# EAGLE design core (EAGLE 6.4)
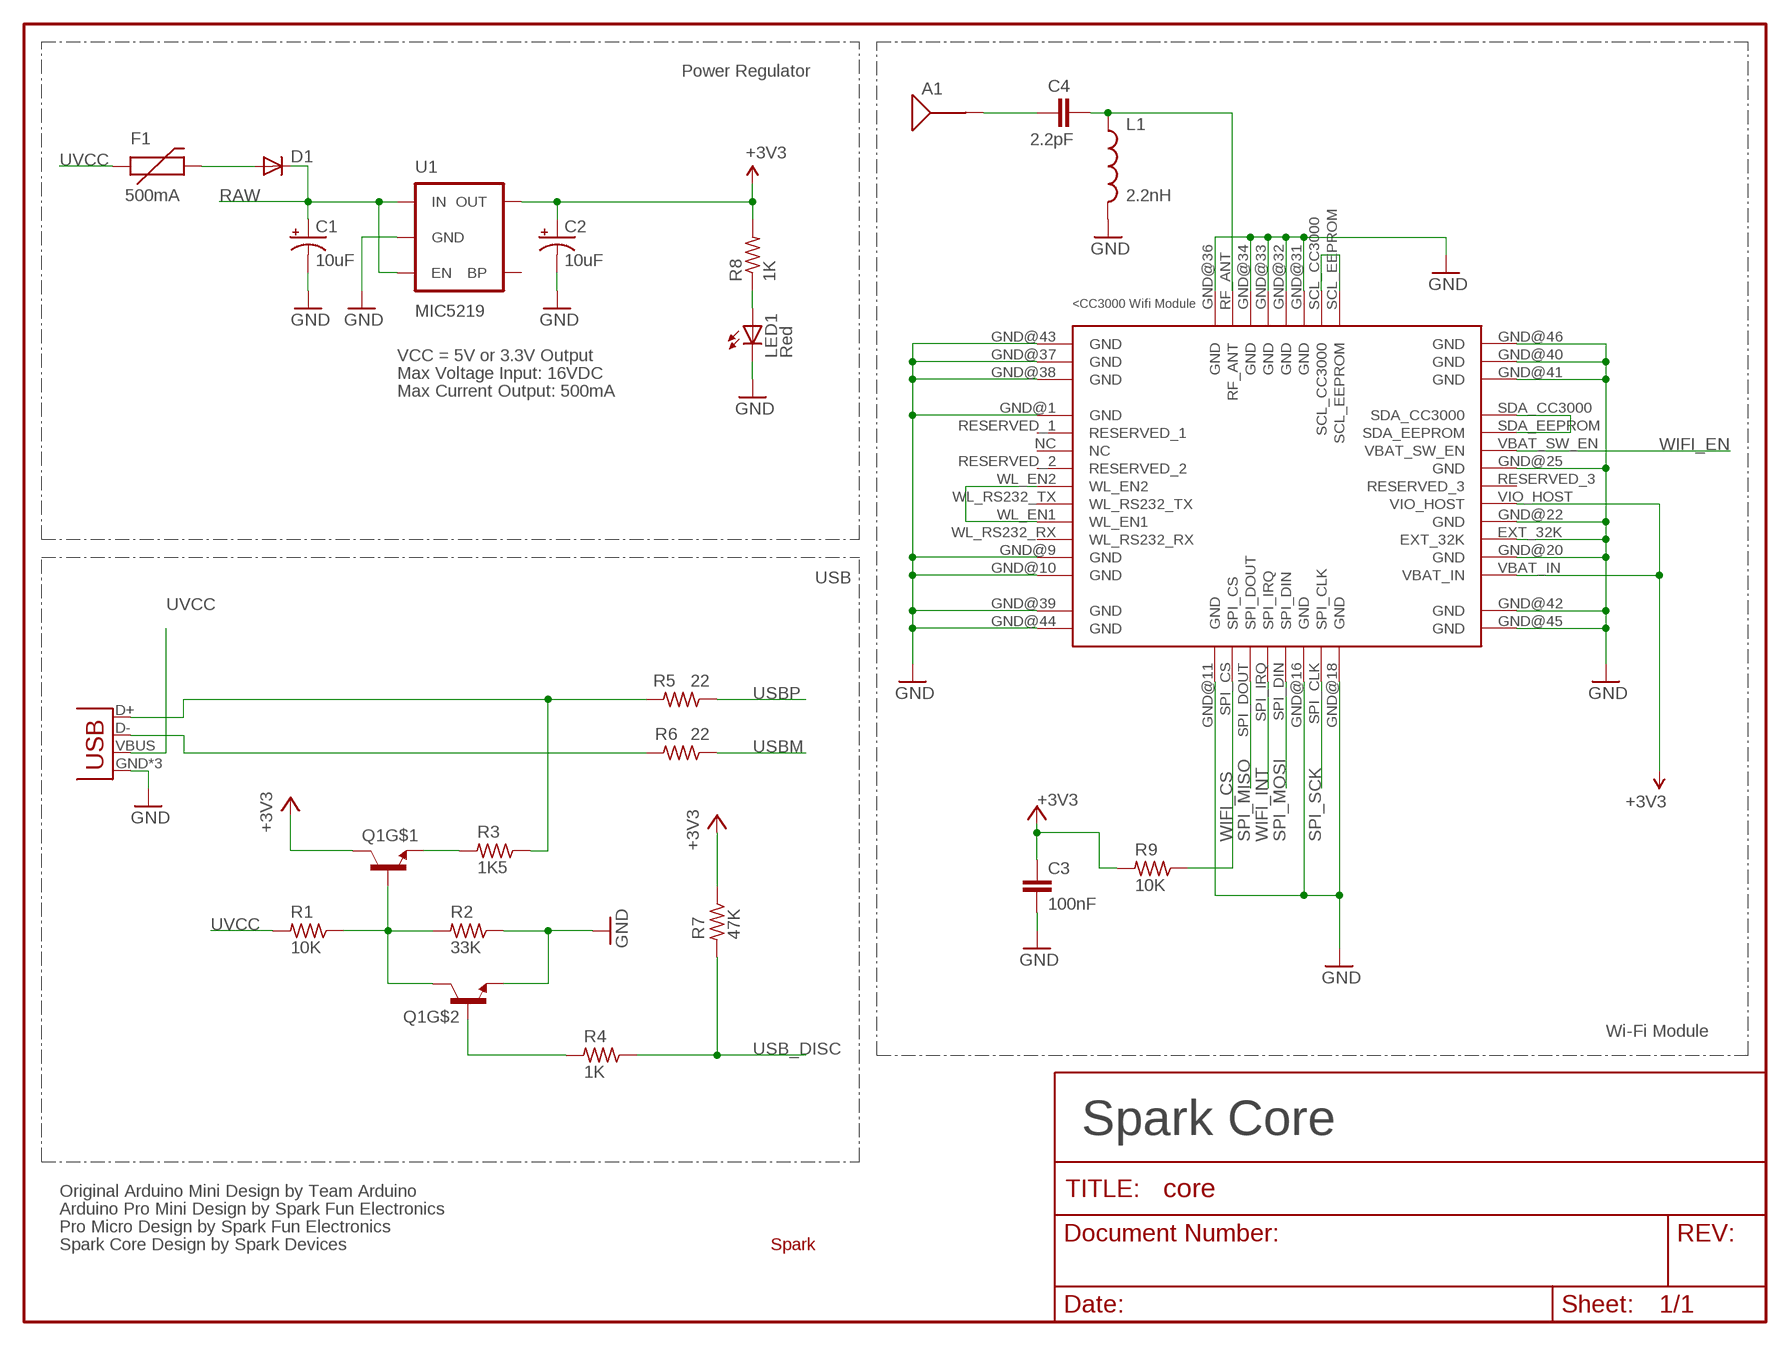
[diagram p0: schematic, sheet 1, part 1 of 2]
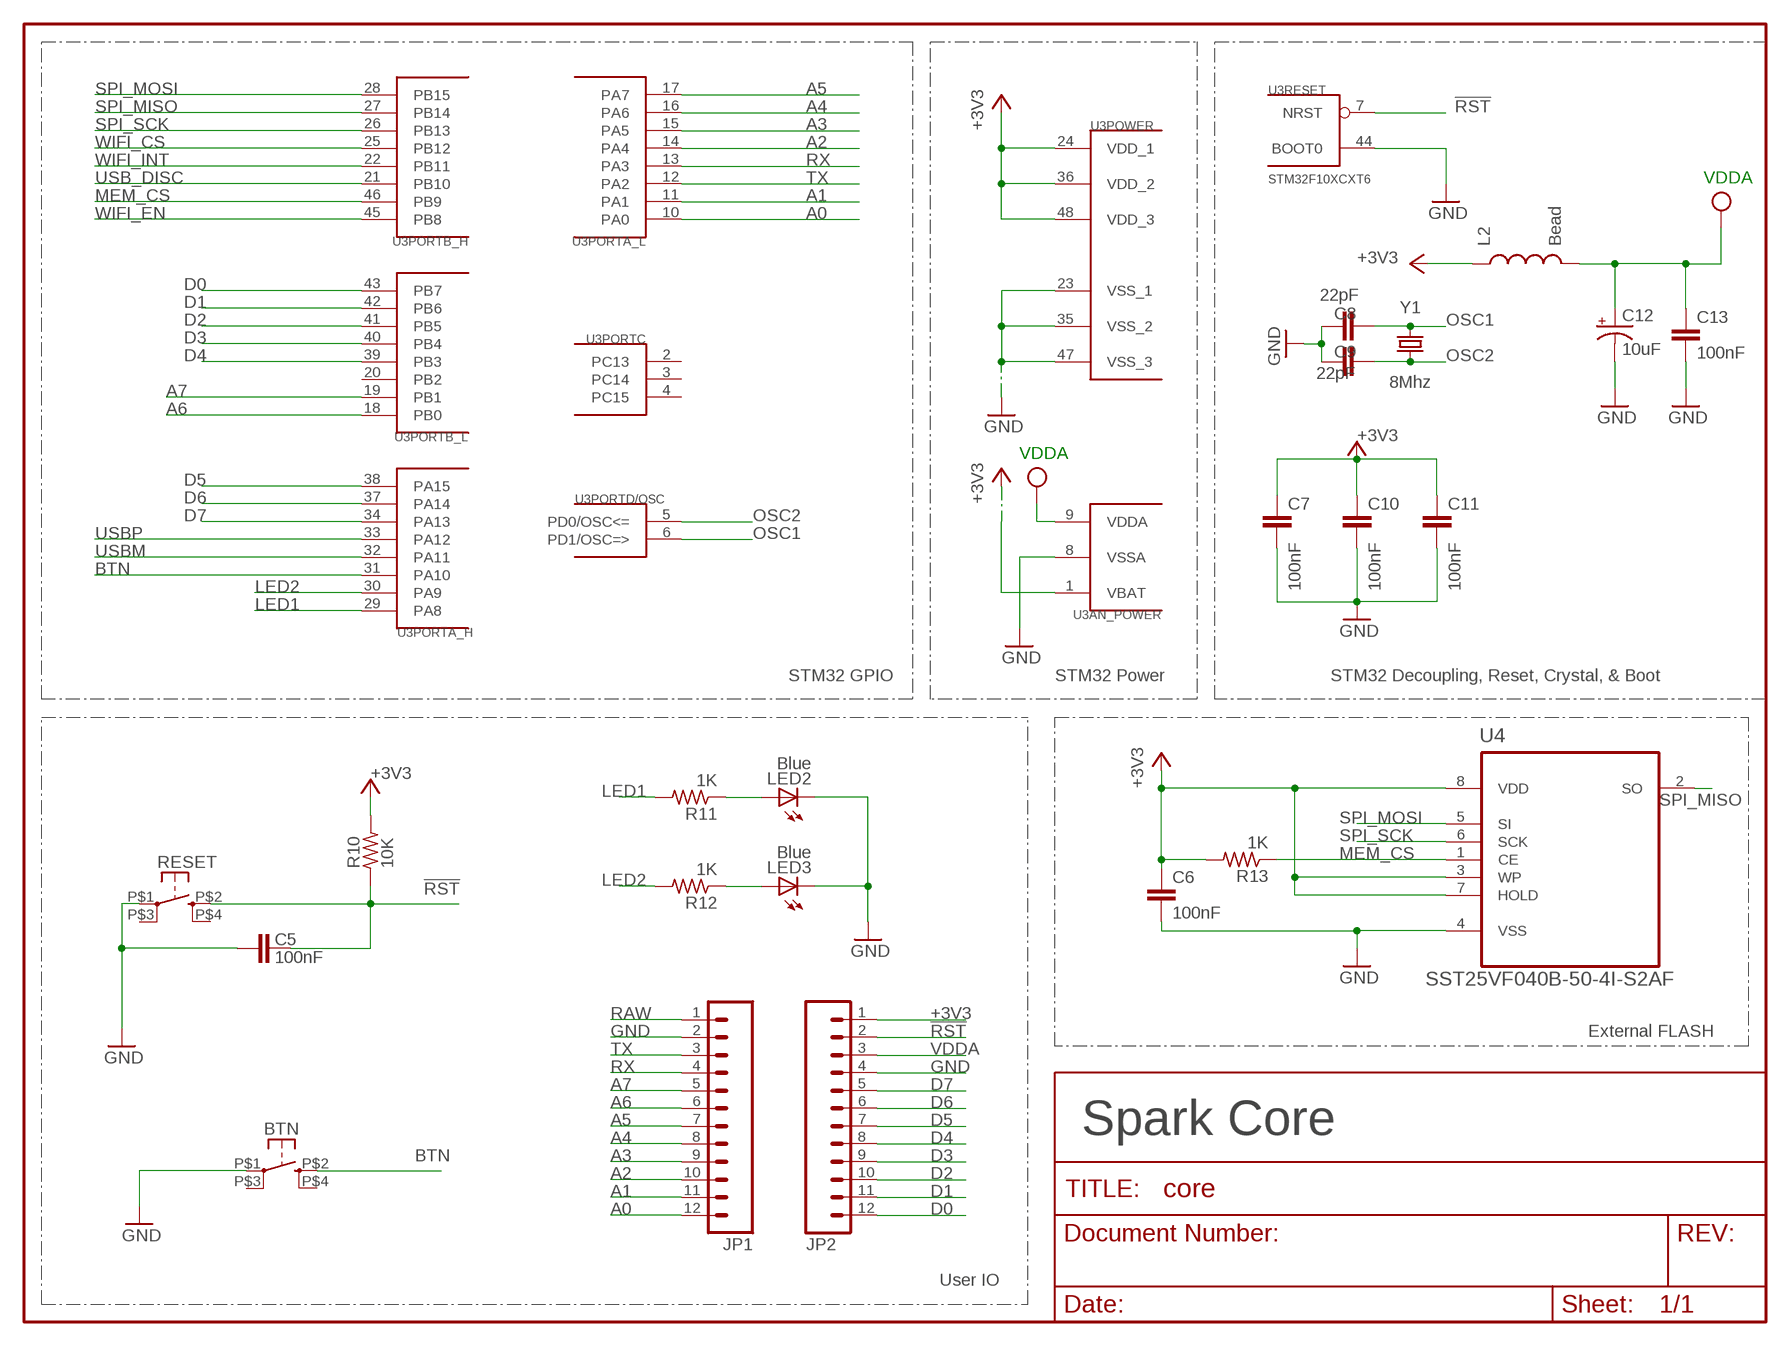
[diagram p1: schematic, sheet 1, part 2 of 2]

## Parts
A1  ANTENNA2SMD5  [ANTENNA-CHIP5]
BTN  KMR211GLFS  BUTTON-KMR241GLFS  [PUSHBUTTON-KMR241GLFS]
C1  10uF  CAP_POL1206  [EIA3216]
C2  10uF  CAP_POL1206  [EIA3216]
C3  100nF  C-EUC0603  [C0603]
C4  2.2pF  C-EUC0603  [C0603]
C5  100nF  C-EUC0603  [C0603]
C6  100nF  C-EUC0603  [C0603]
C7  100nF  C-EUC0603  [C0603]
C8  22pF  C-EUC0603  [C0603]
C9  22pF  C-EUC0603  [C0603]
C10  100nF  C-EUC0603  [C0603]
C11  100nF  C-EUC0603  [C0603]
C12  10uF  CAP_POL1206  [EIA3216]
C13  100nF  C-EUC0603  [C0603]
D1  DIODESOD  [SOD-323]
F1  500mA  PTCSMD  [PTC-1206]
JP1  M12PTH  [1X12]
JP2  M12PTH  [1X12]
L1  2.2nH  INDUCTOR0603  [0603]
L2  Bead  INDUCTOR0603  [0603]
LED1  Red  LED0603  [LED-0603]
LED2  Blue  LED0603  [LED-0603]
LED3  Blue  LED0603  [LED-0603]
Q1  MMDT3904  [SOT363]
R1  10K  R-US_R0603  [R0603]
R2  33K  R-US_R0603  [R0603]
R3  1K5  R-US_R0603  [R0603]
R4  1K  R-US_R0603  [R0603]
R5  22  R-US_R0603  [R0603]
R6  22  R-US_R0603  [R0603]
R7  47K  R-US_R0603  [R0603]
R8  1K  R-US_R0603  [R0603]
R9  10K  R-US_R0603  [R0603]
R10  10K  R-US_R0603  [R0603]
R11  1K  R-US_R0603  [R0603]
R12  1K  R-US_R0603  [R0603]
R13  1K  R-US_R0603  [R0603]
RESET  KMR211GLFS  BUTTON-KMR241GLFS  [PUSHBUTTON-KMR241GLFS]
U1  MIC5219  V_REG_LDOSMD  [SOT23-5]
U2  CC3000  [CC3000]
U3  STM32F10XCXT6  [TQFP48]
U4  SST25VF040B-50-4I-S2AF  [SOIC127P790X216-8N]
U$1  SPARK_LOGO2  [SPARK_LOGO2]
X1  USB-MICROB  USBUSB-MICROB-ALIGN  [USB-MICROB-ALIGN]
Y1  8Mhz  CRYSTAL5X3  [CRYSTAL-SMD-5X3]

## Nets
!RST: C5.2 JP2.2 R10.1 RESET.P$2 U3.7(RESET:NRST)
+3V3: C2.A(+) C3.1 C6.1 C7.1 C10.1 C11.1 JP2.1 L2.1 Q1.3(C) R7.1 R8.2 R9.2 R10.2 R13.2 U1.5(OUT) U2.VBAT_IN U2.VIO_HOST U3.1(AN_POWER:VBAT) U3.24(POWER:VDD_1) U3.36(POWER:VDD_2) U3.48(POWER:VDD_3) U4.3(WP) U4.7(HOLD) U4.8(VDD)
A0: JP1.12 U3.10(PORTA_L:PA0)
A1: JP1.11 U3.11(PORTA_L:PA1)
A2: JP1.10 U3.14(PORTA_L:PA4)
A3: JP1.9 U3.15(PORTA_L:PA5)
A4: JP1.8 U3.16(PORTA_L:PA6)
A5: JP1.7 U3.17(PORTA_L:PA7)
A6: JP1.6 U3.18(PORTB_L:PB0)
A7: JP1.5 U3.19(PORTB_L:PB1)
BTN: BTN.P$2 U3.31(PORTA_H:PA10)
D0: JP2.12 U3.43(PORTB_L:PB7)
D1: JP2.11 U3.42(PORTB_L:PB6)
D2: JP2.10 U3.41(PORTB_L:PB5)
D3: JP2.9 U3.40(PORTB_L:PB4)
D4: JP2.8 U3.39(PORTB_L:PB3)
D5: JP2.7 U3.38(PORTA_H:PA15)
D6: JP2.6 U3.37(PORTA_H:PA14)
D7: JP2.5 U3.34(PORTA_H:PA13)
GND [vcc]: BTN.P$1 C1.C(-) C2.C(-) C3.2 C5.1 C6.2 C7.2 C8.2 C9.2 C10.2 C11.2 C12.C(-) C13.2 JP1.2 JP2.4 L1.2 LED1.C LED2.C LED3.C Q1.1(E) R2.1 RESET.P$1 U1.2(GND) U2.EXT_32K U2.GND@1(GND) U2.GND@9(GND) U2.GND@10(GND) U2.GND@11(GND) U2.GND@16(GND) U2.GND@18(GND) U2.GND@20(GND) U2.GND@22(GND) U2.GND@25(GND) U2.GND@31(GND) U2.GND@32(GND) U2.GND@33(GND) U2.GND@34(GND) U2.GND@36(GND) U2.GND@37(GND) U2.GND@38(GND) U2.GND@39(GND) U2.GND@40(GND) U2.GND@41(GND) U2.GND@42(GND) U2.GND@43(GND) U2.GND@44(GND) U2.GND@45(GND) U2.GND@46(GND) U3.8(AN_POWER:VSSA) U3.23(POWER:VSS_1) U3.35(POWER:VSS_2) U3.44(RESET:BOOT0) U3.47(POWER:VSS_3) U4.4(VSS) X1.GND X1.MT1(GND) X1.MT2(GND)
LED1: R11.2 U3.29(PORTA_H:PA8)
LED2: R12.2 U3.30(PORTA_H:PA9)
MEM_CS: R13.1 U3.46(PORTB_H:PB9) U4.1(CE)
N$1: R3.1 R5.2 X1.D+
N$2: LED2.A R11.1
N$3: D1.2(A) F1.2
N$4: C4.2 L1.1 U2.RF_ANT
N$5: A1.FEED(SIGNAL) C4.1
N$6: R6.2 X1.D-
N$7: U2.SCL_CC3000 U2.SCL_EEPROM
N$8: Q1.2(B) R4.2
N$9: U2.WL_EN1 U2.WL_EN2
N$10: LED3.A R12.1
N$13: Q1.5(B) Q1.6(C) R1.1 R2.2
N$15: U2.SDA_CC3000 U2.SDA_EEPROM
N$16: Q1.4(E) R3.2
N$38: LED1.A R8.1
OSC1: C8.1 U3.6(PORTD/OSC:PD1/OSC=>) Y1.3
OSC2: C9.1 U3.5(PORTD/OSC:PD0/OSC<=) Y1.1
RAW [vcc]: C1.A(+) D1.1(C) JP1.1 U1.1(IN) U1.3(EN)
RX: JP1.4 U3.13(PORTA_L:PA3)
SPI_MISO: U2.SPI_DOUT U3.27(PORTB_H:PB14) U4.2(SO)
SPI_MOSI: U2.SPI_DIN U3.28(PORTB_H:PB15) U4.5(SI)
SPI_SCK: U2.SPI_CLK U3.26(PORTB_H:PB13) U4.6(SCK)
TX: JP1.3 U3.12(PORTA_L:PA2)
USB_DISC: R4.1 R7.2 U3.21(PORTB_H:PB10)
USBM: R6.1 U3.32(PORTA_H:PA11)
USBP: R5.1 U3.33(PORTA_H:PA12)
UVCC: F1.1 R1.2 X1.VBUS
VDDA: C12.A(+) C13.1 JP2.3 L2.2 U3.9(AN_POWER:VDDA) ; supply symbol labelled VCC
WIFI_CS: R9.1 U2.SPI_CS U3.25(PORTB_H:PB12)
WIFI_EN: U2.VBAT_SW_EN U3.45(PORTB_H:PB8)
WIFI_INT: U2.SPI_IRQ U3.22(PORTB_H:PB11)
Unconnected: BTN.P$3 BTN.P$4 RESET.P$3 RESET.P$4 U1.4(BP) U2.NC U2.RESERVED_1 U2.RESERVED_2 U2.RESERVED_3 U2.WL_RS232_RX U2.WL_RS232_TX U3.2(PORTC:PC13) U3.3(PORTC:PC14) U3.4(PORTC:PC15) U3.20(PORTB_L:PB2)

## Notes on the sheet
- Power Regulator
- VDDA
- VCC = 5V or 3.3V Output
- Max Voltage Input: 16VDC
- Max Current Output: 500mA
- VDDA
- USB
- STM32 GPIO | STM32 Power | STM32 Decoupling, Reset, Crystal, & Boot
- Wi-Fi Module | External FLASH
- Spark Core | Spark Core
- Original Arduino Mini Design by Team Arduino
- Arduino Pro Mini Design by Spark Fun Electronics
- Pro Micro Design by Spark Fun Electronics
- Spark Core Design by Spark Devices
- User IO

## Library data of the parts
A1 = SparkFun-RF:ANTENNA2: Chip antenna
BTN RESET = okie:BUTTON-KMR241GLFS
C1 C2 C12 = SparkFun:CAP_POL: Capacitor Polarized
C3-C11 C13 = rcl:C-EU: CAPACITOR, European symbol
D1 = SparkFun:DIODE: Diode
F1 = SparkFun:PTC: Resettable Fuse PTC
JP1 JP2 = SparkFun:M12: Header 12 Standard 12-pin 0.1" header. Use with straight break away headers (SKU : PRT-00116), right angle break away headers (PRT-00553), swiss pins (PRT-00743), machine pins (PRT-00117), and female headers (PRT-00115).
L1 L2 = SparkFun-Passives:INDUCTOR: Inductors
LED1-LED3 = SparkFun:LED: LEDs
Q1 = SparkFun-DiscreteSemi:MMDT3904: Dual NPN transistor
R1-R13 = rcl:R-US_: RESISTOR, American symbol
U1 = SparkFun:V_REG_LDO: Voltage Regulator LDO Standard 150mA LDO voltage regulator in SOT-23 layout. Micrel part MIC5205. BP (by-pass) pin is used to lower output noise with 470pF cap.
U2 = CC3000:CC3000
U3 = stm32:STM32F10XCXT6: ST STM32F101/103 48pin LQFP
U4 = Silicon_Storage_Tech_By_element14_Batch_1:SST25VF040B-50-4I-S2AF: 4 Mbit SPI Serial Flash; MPN: SST25VF040B-50-4I-S2AF; OC_FARNELL: 1368690; OC_NEWARK: -; PACKAGE: SOIC-8; SUPPLIER: SILICON STORAGE TECHNOLOGY
U$1 = Spark:SPARK_LOGO2
X1 = Spark:USB: USB Connectors USB-B-PTH is fully proven SKU : PRT-00139/CONN-08278 USB-miniB is fully proven SKU : PRT-00587 USB-A-PCB is untested. USB-A-H is throughly reviewed, but untested. Spark Fun Electronics SKU : PRT-00437 USB-B-SMT is throughly reviewed, but untested. Needs silkscreen touching up.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
Y1 = SparkFun:CRYSTAL: Crystals

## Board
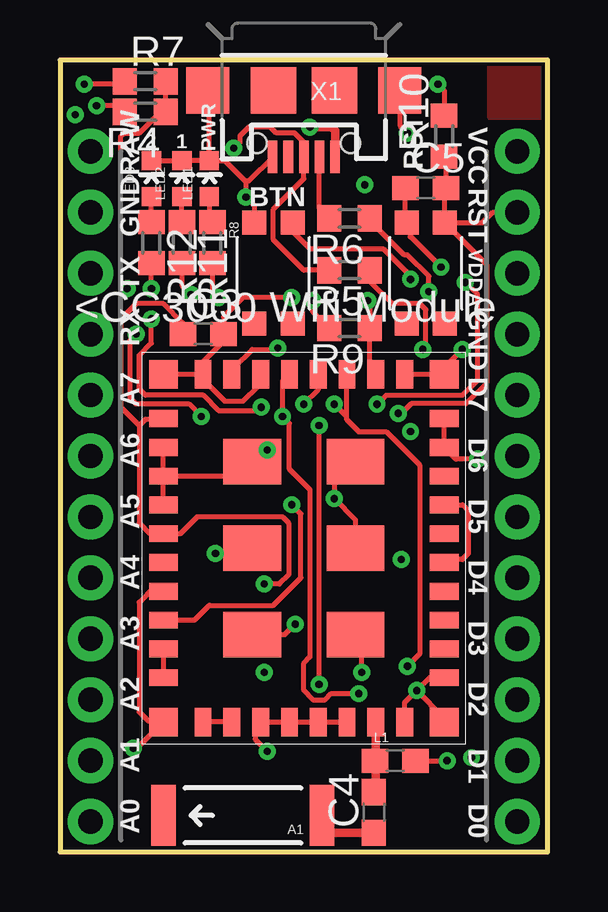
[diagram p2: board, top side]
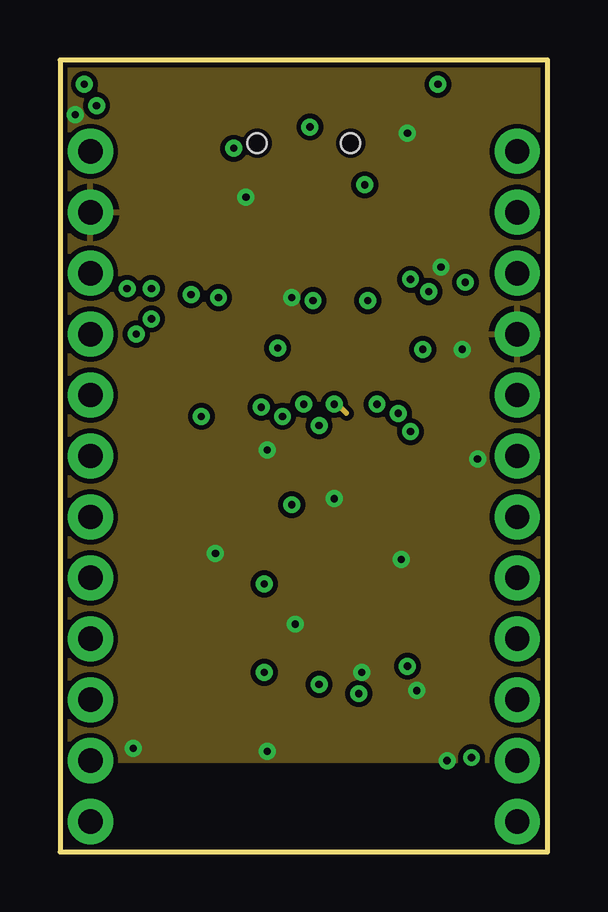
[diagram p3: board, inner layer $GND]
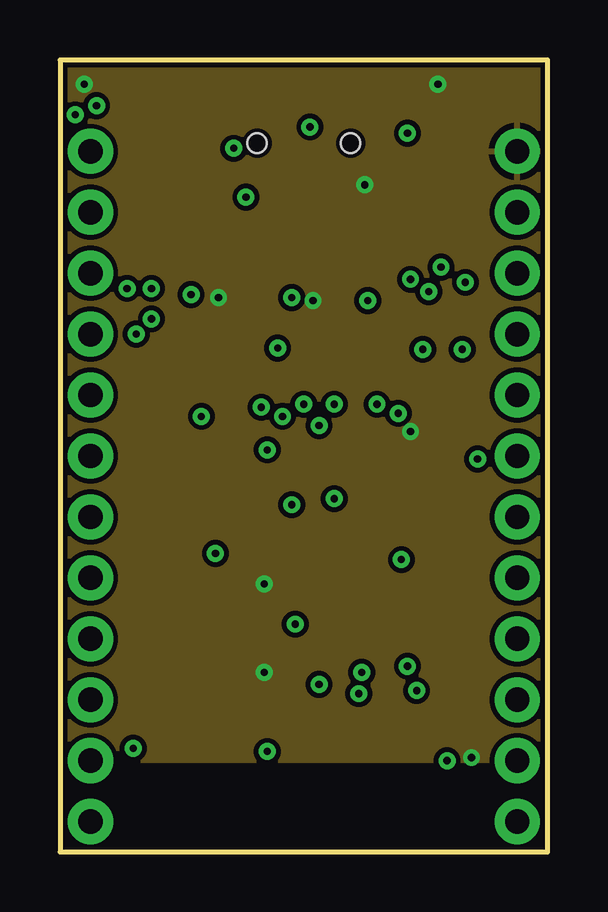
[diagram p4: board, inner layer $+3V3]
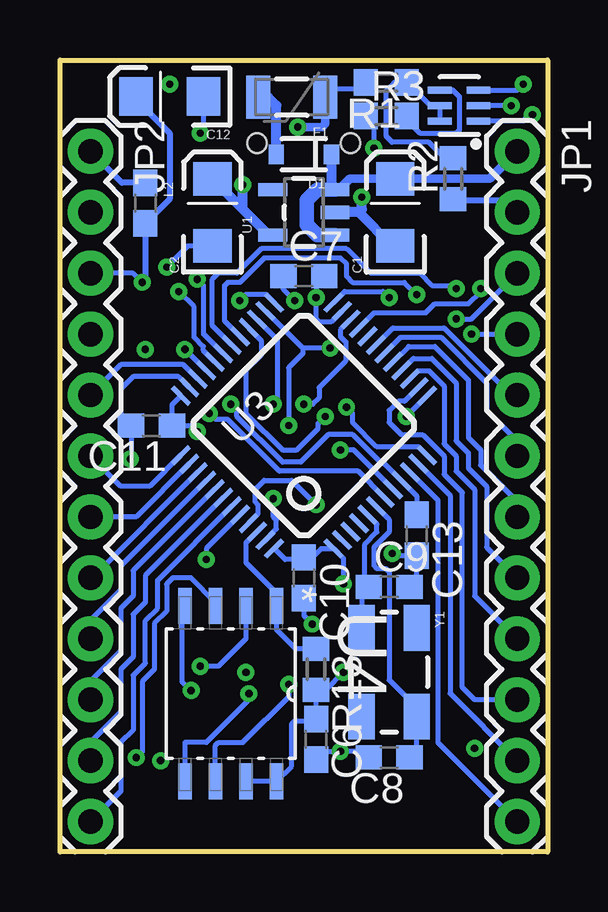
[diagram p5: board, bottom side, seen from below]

Size 20.32 x 33.02 mm. Coordinates in mm from the lower left corner, seen from the top.
Outline: 0,33.02 0,0 20.32,0 20.32,33.02 0,33.02
Copper layers (1+2*15+16): Top 0.035mm / dielectric 1.5mm / $GND 0.035mm / dielectric 0.15mm / $+3V3 0.035mm / dielectric 0.2mm / Bottom 0.035mm
Design rules "default *": minimum track width 6mil, minimum drill 0.3mm, track to track 6mil, track to pad 6mil, pad to pad 6mil, via to via 6mil, smd to smd 6mil, copper to edge 6mil, drill to drill 6mil, minimum pad ring 12mil, minimum via ring 8mil, stop-mask expansion 4mil, vias tented up to drill 20mil, thermal gap 10mil

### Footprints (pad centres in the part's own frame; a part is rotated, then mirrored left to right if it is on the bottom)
ANTENNA-CHIP5 = smd 1.016 x 2.54: FEED -3.302,0; NC 3.302,0
PUSHBUTTON-KMR241GLFS = smd 1 x 1: P$1 2.1,0.8; P$2 2.1,-0.8; P$3 -2.1,0.8; P$4 -2.1,-0.8
EIA3216 = smd 1.4 x 1.6: A 1.4,0; C -1.4,0
C0603 = smd 1.1 x 1: 1 -0.85,0; 2 0.85,0
SOD-323 = smd 0.63 x 0.83: 1 -1.15,0; 2 1.15,0
PTC-1206 = smd 1 x 1.8: 1 -1.4,0; 2 1.4,0
1X12 = drill 1.016 pad 1.88: 1 0,0; 2 2.54,0; 3 5.08,0; 4 7.62,0; 5 10.16,0; 6 12.7,0; 7 15.24,0; 8 17.78,0; 9 20.32,0; 10 22.86,0; 11 25.4,0; 12 27.94,0
0603 = smd 1.1 x 1: 1 -0.85,0; 2 0.85,0
LED-0603 = smd 0.8 x 0.8: A 0,-0.75; C 0,0.75
SOT363 = smd 0.3 x 0.99: 1 -0.65,-0.8; 2 0,-0.8; 3 0.65,-0.8; 4 0.65,0.81; 5 0,0.81; 6 -0.65,0.81
R0603 = smd 1 x 1.1: 1 -0.85,0; 2 0.85,0
SOT23-5 = smd 0.55 x 1.2: 1 -0.95,-1.3; 2 0,-1.3; 3 0.95,-1.3; 4 0.95,1.3; 5 -0.95,1.3
CC3000 = smd 1.2 x 0.7: EXT_32K 5.85,-2.97; GND@1 -5.85,5.43; GND@9 -5.85,-4.17; GND@10 -5.85,-5.37; GND@20 5.85,-4.17; GND@22 5.85,-1.77; GND@25 5.85,1.83; NC -5.85,3.03; RESERVED_1 -5.85,4.23; RESERVED_2 -5.85,1.83; RESERVED_3 5.85,0.63; SDA_CC3000 5.85,5.43; SDA_EEPROM 5.85,4.23; VBAT_IN 5.85,-5.37; VBAT_SW_EN 5.85,3.03; VIO_HOST 5.85,-0.57; WL_EN1 -5.85,-1.77; WL_EN2 -5.85,0.63; WL_RS232_RX -5.85,-2.97; WL_RS232_TX -5.85,-0.57 | smd 0.7 x 1.2: GND@11 -4.2,-7.22; GND@16 1.8,-7.22; GND@18 4.2,-7.22; GND@31 1.8,7.28; GND@32 0.6,7.28; GND@33 -0.6,7.28; GND@34 -1.8,7.28; GND@36 -4.2,7.28; RF_ANT -3,7.28; SCL_CC3000 3,7.28; SCL_EEPROM 4.2,7.28; SPI_CLK 3,-7.22; SPI_CS -3,-7.22; SPI_DIN 0.6,-7.22; SPI_DOUT -1.8,-7.22; SPI_IRQ -0.6,-7.22 | smd 2.4 x 1.9: GND@37 -2.15,3.63; GND@38 -2.15,0.03; GND@39 -2.15,-3.57; GND@40 2.15,3.63; GND@41 2.15,0.03; GND@42 2.15,-3.57 | smd 1.2 x 1.2: GND@43 -5.85,7.28; GND@44 -5.85,-7.22; GND@45 5.85,-7.22; GND@46 5.85,7.28
TQFP48 = smd 0.2 x 1: 1 -2.75,-4.5; 2 -2.25,-4.5; 3 -1.75,-4.5; 4 -1.25,-4.5; 5 -0.75,-4.5; 6 -0.25,-4.5; 7 0.25,-4.5; 8 0.75,-4.5; 9 1.25,-4.5; 10 1.75,-4.5; 11 2.25,-4.5; 12 2.75,-4.5; 25 2.75,4.5; 26 2.25,4.5; 27 1.75,4.5; 28 1.25,4.5; 29 0.75,4.5; 30 0.25,4.5; 31 -0.25,4.5; 32 -0.75,4.5; 33 -1.25,4.5; 34 -1.75,4.5; 35 -2.25,4.5; 36 -2.75,4.5 | smd 1 x 0.2: 13 4.5,-2.75; 14 4.5,-2.25; 15 4.5,-1.75; 16 4.5,-1.25; 17 4.5,-0.75; 18 4.5,-0.25; 19 4.5,0.25; 20 4.5,0.75; 21 4.5,1.25; 22 4.5,1.75; 23 4.5,2.25; 24 4.5,2.75; 37 -4.5,2.75; 38 -4.5,2.25; 39 -4.5,1.75; 40 -4.5,1.25; 41 -4.5,0.75; 42 -4.5,0.25; 43 -4.5,-0.25; 44 -4.5,-0.75; 45 -4.5,-1.25; 46 -4.5,-1.75; 47 -4.5,-2.25; 48 -4.5,-2.75
SOIC127P790X216-8N = smd 1.499 x 0.559: 1 -3.658,1.905; 2 -3.658,0.635; 3 -3.658,-0.635; 4 -3.658,-1.905; 5 3.658,-1.905; 6 3.658,-0.635; 7 3.658,0.635; 8 3.658,1.905
USB-MICROB-ALIGN = smd 0.4 x 1.35: D+ 0,2.775; D- -0.65,2.775; GND 1.3,2.775; ID 0.65,2.775; VBUS -1.3,2.775 | smd 1.8 x 1.95: MT1 -4,0; MT2 4,0 | smd 1.9 x 1.95: P$1 -1.27,0; P$2 1.27,0 | hole 0.8: -1.95,2.2; 1.95,2.2
CRYSTAL-SMD-5X3 = smd 1.9 x 1.1: 1 -1.85,-1.15; 2 1.85,-1.15; 3 1.85,1.15; 4 -1.85,1.15

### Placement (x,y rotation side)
A1  7.62,1.52 180 top
BTN  8.89,24.13 90 top
C1  6.35,26.67 90 bottom
C2  13.97,26.67 90 bottom
C3  5.97,21.59 0 top
C4  13.08,1.65 90 top
C5  15.24,27.69 0 top
C6  9.65,4.7 270 bottom
C7  10.16,24 0 bottom
C8  6.6,3.94 180 bottom
C9  6.6,11.05 0 bottom
C10  10.16,11.43 270 bottom
C11  16.51,17.78 180 bottom
C12  15.75,31.5 180 bottom
C13  5.46,13.21 270 bottom
D1  10.16,29.08 180 bottom
F1  10.67,31.47 180 bottom
JP1  1.27,29.21 270 bottom
JP2  19.05,29.21 270 bottom
L1  13.97,3.81 0 top
L2  16.76,27.05 270 bottom
LED1  6.22,28.07 0 top
LED2  5.08,28.07 0 top
LED3  3.81,28.07 0 top
Q1  3.68,31.11 90 bottom
R1  6.73,32.08 180 bottom
R2  3.94,28.07 90 bottom
R3  6.73,30.68 0 bottom
R4  3.56,30.86 180 top
R5  12.06,24.26 180 top
R6  12.06,26.42 180 top
R7  3.56,32.13 0 top
R8  6.35,25.4 270 top
R9  12.06,21.84 180 top
R10  16,29.84 90 top
R11  5.08,25.4 270 top
R12  3.81,25.4 270 top
R13  9.65,7.62 270 bottom
RESET  15.24,24.13 90 top
U1  10.16,26.67 90 bottom
U2  10.16,12.7 180 top
U3  10.16,17.78 45 bottom
U4  13.21,6.6 270 bottom
U$1  17.78,30.48 0 top
X1  10.16,31.75 180 top
Y1  6.6,7.49 270 bottom

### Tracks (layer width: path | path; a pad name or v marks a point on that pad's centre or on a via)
!RST  (via drill 0.3)
  Top 0.203: JP2.2 18.03,26.67 17.59,26.23 RESET.P$2 | RESET.P$2 17.78,24.49 17.78,19.56 16.92,18.69 14.63,18.69 14.22,18.29 v14.1,18.29 | RESET.P$2 16.04,27.64 C5.2 16.09,28.91 R10.1
  Bottom 0.203: U3.7 7.9,15.88 11.18,15.88 13.34,18.03 13.84,18.03 v14.1,18.29
+3V3  (via drill 0.3)
  Top 0.203: U2.VBAT_IN 4.27,18.03 3.56,18.03 3.3,17.78 | 3.3,17.78 3.3,13.72 3.75,13.27 U2.VIO_HOST 5.01,13.27 5.71,13.97 9.27,13.97 9.53,13.72 9.53,11.56 9.14,11.18 v8.51,11.18 | R9.2 10.54,22.52 v10.54,22.99 | v15.75,32 16,31.75 R10.2 | R7.1 2.58,32 v1.02,32 | R8.2 6.35,23.37 v6.6,23.11 | C3.1 5.12,22.06 4.32,22.86 3.17,22.86 2.54,22.23 2.54,18.54 3.3,17.78
  Bottom 0.203: C10.1 10.16,12.19 10.94,12.19 U3.48 | 10.16,12.06 C10.1 | 8.97,12.7 U3.1 | C10.1 10.16,11.94 9.45,12.65 U3.1 | U3.24 8.46,23.37 6.86,23.37 v6.6,23.11 | U4.7 U4.8 10.67,3.58 10.67,5.33 10.54,5.46 9.74,5.46 C6.1 R13.2 9.23,6.77 v8.51,7.49 | U4.3 13.84,10.41 14.86,11.43 15.62,11.43 15.88,11.18 15.88,10.03 16.38,9.53 16.38,7.62 16.89,7.11 16.89,4.19 v17.14,3.94 | U3.1 8.51,12.24 v8.51,11.18 | U3.36 15.66,18.64 C11.1 14.86,17.78 v14.61,17.53 | v10.54,22.99 11.01,23.46 C7.1 | Q1.3 1.25,31.77 v1.02,32
  Bottom 0.254: L2.1 17.74,27.9 JP2.1
  Bottom 0.406: U1.5 11.62,25.72 12.7,26.8 | 12.7,26.8 v12.7,27.81 | C2.A 12.7,26.8
  pour $+3V3 (isolate 0.203): 0,33.02 20.32,33.02 20.32,3.81 0,3.81
A0
  Bottom 0.203: JP1.12 4.57,4.57 4.57,14.67 U3.10
A1
  Bottom 0.203: JP1.11 4.06,6.6 4.06,14.87 U3.11
A2
  Bottom 0.203: JP1.10 3.05,6.35 3.56,6.86 3.56,14.99 4.32,15.75 4.32,16.51 5.21,17.4 6.1,17.4 6.6,17.91 6.6,18.41 6.22,18.8 5.96,18.8 U3.14
A3
  Bottom 0.203: JP1.9 3.05,10.67 3.05,15.11 3.81,15.88 3.81,16.51 4.32,17.02 4.32,19.43 4.95,20.07 5.4,20.07 U3.15
A4
  Bottom 0.203: U3.16 5.6,20.57 4.83,20.57 3.81,19.56 3.81,17.14 3.3,16.64 3.3,16 2.54,15.24 2.54,12.7 JP1.8
A5
  Bottom 0.203: JP1.7 1.27,14.61 2.79,16.13 2.79,16.76 3.3,17.27 3.3,19.68 4.7,21.08 5.8,21.08 U3.17
A6
  Bottom 0.203: U3.18 6.12,21.46 4.45,21.46 2.54,19.56 2.54,18.41 1.27,17.14 JP1.6
A7
  Bottom 0.203: 1.4,19.05 JP1.5 1.52,19.05 4.32,21.84 6.45,21.84 U3.19
BTN  (via drill 0.3)
  Top 0.203: BTN.P$2 9.69,25.87 10.41,25.15 13.46,25.15 14.61,24 v14.61,23.88
  Bottom 0.203: v14.61,23.88 14.35,23.62 14.35,21.59 14.32,21.59 U3.31
D0
  Bottom 0.203: U3.43 16.26,11.33 16.26,10.16 16.76,9.65 16.76,7.87 17.27,7.37 17.27,5.08 17.78,4.57 17.78,2.54 JP2.12
D1
  Bottom 0.203: JP2.11 19.05,4.57 17.78,5.84 17.78,7.62 17.27,8.13 17.27,9.91 16.76,10.41 16.76,11.53 U3.42
D2
  Bottom 0.203: JP2.10 19.05,7.11 17.78,8.38 17.78,10.16 17.27,10.67 17.27,11.73 U3.41
D3
  Bottom 0.203: JP2.9 19.05,9.65 17.78,10.92 17.78,11.94 17.77,11.94 U3.40
D4
  Bottom 0.203: U3.39 18.98,11.43 JP2.8
D5
  Bottom 0.203: JP2.7 17.15,13.97 U3.38
D6
  Bottom 0.203: U3.37 16.59,15.24 17.78,15.24 JP2.6
D7
  Bottom 0.203: JP2.5 17.78,20.32 15.18,20.32 U3.34
GND  (via drill 0.3)
  Top 0.203: U2.GND@43 16.01,5.58 v14.86,6.73 | U2.GND@36 14.36,6.23 v14.86,6.73 | U2.GND@1 15.4,7.27 v14.86,6.73 | v12.57,7.49 12.57,8.81 U2.GND@37 | 12.06,16.52 U2.GND@39 11.43,15.39 v11.43,14.73 12.31,13.85 U2.GND@38 12.41,12.57 | v8.64,16.76 8.14,16.27 U2.GND@42 7.41,15.67 U2.EXT_32K | U2.GND@31 U2.GND@32 U2.GND@33 U2.GND@34 | 8.36,5.86 U2.GND@31 | U2.GND@41 7.66,12.32 7.53,12.45 v6.48,12.45 | U2.GND@22 U2.EXT_32K | U2.GND@45 U2.GND@18 | U2.GND@10 U2.GND@9 16.5,16.38 v17.4,16.38 | U2.GND@25 4.49,11.05 3.94,11.05 3.3,10.41 3.3,5.84 3.68,5.46 4.27,5.46 U2.GND@46 3.21,4.32 v3.05,4.32 | U2.GND@11 U2.GND@44 16,20.19 v16.76,20.95 | 14.59,26.38 RESET.P$1 | U2.EXT_32K U2.GND@20 | U2.GND@18 | 8.31,26.23 BTN.P$1 8.09,26.96 v7.75,27.3 7.75,27.94 | 14.59,26.38 14.59,25.65 14.61,25.65 v15.88,24.38 | U2.GND@31 8.13,5.19 8.13,4.7 v8.64,4.19 | X1.MT1 14.16,30.29 v14.48,29.97 | U2.GND@40 9.38,9.07 v9.8,9.5 | 7.75,27.94 7.75,27.99 7.87,27.99 X1.GND | 14.59,26.38 14.39,26.58 C5.1 | v9.65,23.11 7.62,23.11 6.82,22.31 C3.2 6.82,21.3 5.96,20.44 U2.GND@18 | U2.GND@18 5.96,19.69 6.86,18.8 7.62,18.8 8.26,19.43 8.26,19.82 U2.GND@16 | 5.96,20.31 U2.GND@18 | L1.2 v16.13,3.81 | LED3.C LED2.C LED1.C | LED1.C 6.87,28.82 7.75,27.94 | LED1.C 6.22,31.69 X1.MT2
  Top 0.254: X1.MT2 6.21,31.75
  Bottom 0.203: U3.35 15.37,19.81 17.27,19.81 17.78,19.3 17.78,18.2 C11.2 17.36,16.42 v17.4,16.38 | U3.47 11.8,12.95 11.81,12.95 11.3,13.46 11.3,13.84 11.43,13.97 v11.43,14.73 | U3.8 8.08,16.76 v8.64,16.76 | U4.4 15.24,10.13 15.24,7.11 v14.86,6.73 | C6.2 9.65,4.19 v8.64,4.19 7.71,4.19 C8.2 | C12.C 14.35,30.1 v14.48,29.97 | C10.2 10.16,9.86 v9.8,9.5 | C9.2 5.46,11.34 C13.2 6.39,12.36 v6.48,12.45 | U3.44 14.22,12.65 v14.22,12.19 | C7.2 9.65,23.66 v9.65,23.11 9.65,22.23 9.53,22.1 9.02,22.1 U3.23 | C2.C 14.99,25.27 v15.88,24.38 | Q1.1 2.87,30.48 1.02,30.48 0.76,30.73 v0.64,30.73
  Bottom 0.254: R2.1 3.9,27.18 1.78,27.18 JP1.2
  Bottom 0.406: 7.87,26.67 U1.2 | 7.87,26.67 7.75,26.8 v7.75,27.3 | C1.C 6.47,25.27 7.87,26.67
  pour $GND (isolate 0.203): 0,33.02 20.32,33.02 20.32,3.81 0,3.81
LED1  (via drill 0.3)
  Top 0.203: R11.2 5.08,23.62 v5.46,23.24
  Bottom 0.203: U3.29 13.46,22.14 13.46,23.62 13.34,23.75 12.83,23.75 11.81,24.77 8.64,24.77 8.38,24.51 8.38,24 8.13,23.75 5.97,23.75 v5.46,23.24
LED2  (via drill 0.3)
  Top 0.203: v3.81,23.5 R12.2
  Bottom 0.203: U3.30 13.97,21.94 13.97,23.88 13.72,24.13 12.95,24.13 11.94,25.15 8.38,25.15 7.37,24.13 5.33,24.13 4.83,23.62 3.94,23.62 v3.81,23.5
MEM_CS
  Bottom 0.203: R13.1 10.5,8.47 11.3,9.27 U4.1 11.3,10.79 12.57,12.06 12.57,12.89 U3.46
N$1  (via drill 0.3)
  Top 0.203: R5.2 10.16,24.26 8.89,25.53 8.89,26.8 10.16,28.07 X1.D+ 10.16,29.59 9.78,29.97 9.02,29.97 8.76,30.23 7.87,30.23 7.49,29.84 7.49,29.59 v7.24,29.34
  Bottom 0.203: v7.24,29.34 7.24,30.21 7.49,30.47 7.49,30.73 7.87,30.35 7.87,30.23 7.58,30.52 R3.1
N$2
  Top 0.203: R11.1 LED2.A
N$3
  Bottom 0.203: F1.2 12.04,31.47
  Bottom 0.356: D1.2
  Bottom 0.406: D1.2 11.3,31.11 11.66,31.47 F1.2
N$4
  Top 0.363: U2.RF_ANT 13.16,3.68 | 13.16,3.68 13.16,2.58 C4.2 | L1.1 13.12,3.72 13.16,3.68
N$5
  Top 0.363: C4.1 10.96,0.8 10.92,0.76 A1.FEED
N$6
  Top 0.203: R6.2 10.81,26.82 X1.D-
N$7
  Top 0.203: U2.SCL_CC3000 U2.SCL_EEPROM
N$8  (via drill 0.3)
  Top 0.203: R4.2 2.45,31.11 v1.52,31.11
  Bottom 0.203: v1.52,31.11 Q1.2
N$9
  Top 0.203: U2.WL_EN1 16.77,14.47 17.02,14.22 17.02,12.45 16.76,12.19 16.13,12.19 U2.WL_EN2
N$10
  Top 0.203: R12.1 LED3.A
N$11
  pour Top: 17.91,33.02 20.32,33.02 20.32,30.61 17.91,30.61
N$13
  Bottom 0.203: Q1.6 Q1.5 4.9,31.11 5.87,32.08 R1.1 | R2.2 4.28,28.92 4.95,29.59 6.48,29.59 6.73,29.84 6.73,31.75 6.4,32.08 R1.1 | 5.96,32 R1.1
N$15
  Top 0.203: U2.SDA_EEPROM U2.SDA_CC3000
N$16
  Bottom 0.203: Q1.4 3.95,31.77 3.68,31.5 3.68,30.1 3.81,29.97 5.33,29.97 5.59,30.23 5.59,30.39 R3.2
N$38
  Top 0.203: LED1.A 6.22,26.38 R8.1
OSC1
  Bottom 0.203: U3.6 6.6,13.87 6.6,13.34 7.24,12.7 7.24,11.94 7.11,11.81 6.73,11.81 6.6,11.68 6.6,7.17 5.45,6.02 Y1.3 5.45,4.24 C8.1
OSC2
  Bottom 0.203: U3.5 7.11,13.67 7.11,13.34 7.62,12.83 7.62,11.21 C9.1 7.75,10.75 Y1.1
RAW
  Bottom 0.203: 8.93,27.69 U1.3 9.01,27.77
  Bottom 0.356: JP1.1 2.41,28.07 C1.A 7.88,28.07 8.26,28.07 8.7,27.62 U1.3
  Bottom 0.406: D1.1 9.01,27.77
  Bottom 0.61: U1.3 9.59,27.62 10.03,27.18 10.03,26.16 9.59,25.72 U1.1
RX  (via drill 0.3)
  Top 0.203: v5.89,18.16 5.36,18.69 3.15,18.69 2.92,18.92 2.92,21.34 v3.17,21.59
  Bottom 0.203: U3.13 v5.89,18.16 | v3.17,21.59 JP1.4
SPI_MISO  (via drill 0.3)
  Top 0.203: v14.48,7.75 14.99,8.26 14.99,16.13 13.59,17.53 12.45,17.53 11.94,18.03 11.94,18.16 | 11.94,18.16 11.94,19.9 U2.SPI_DOUT | 11.94,18.16 v11.43,18.67
  $GND 0.203: v11.43,18.67 11.56,18.67 11.94,18.29
  Bottom 0.203: U4.2 12.57,8.89 13.72,7.75 v14.48,7.75 | U3.27 11.28,21.37 11.28,18.82 v11.43,18.67
SPI_MOSI  (via drill 0.3)
  Top 0.203: v12.45,6.6 11.3,6.6 11.05,6.35 10.54,6.35 10.16,6.73 10.16,7.87 10.41,8.13 10.41,15.11 9.56,15.97 9.56,17.87 v9.27,18.16 9.27,19.63 U2.SPI_DIN
  Bottom 0.203: U4.5 15.11,4.57 14.22,4.57 12.45,6.35 v12.45,6.6 | U3.28 11.94,21.33 11.94,20.7 12.57,20.07 12.57,18.29 11.05,16.76 10.45,16.76 9.56,17.65 9.56,17.87 v9.27,18.16
SPI_SCK  (via drill 0.3)
  Top 0.203: 7.16,20.37 U2.SPI_CLK 7.24,20 7.24,20.19 8,20.95 9.02,20.95 v9.07,21.01 | v10.79,6.99 v10.79,17.78
  Bottom 0.203: U4.6 13.84,4.45 13.72,4.57 12.7,4.57 10.79,6.48 v10.79,6.99 | U3.26 10.2,21.01 | v9.07,21.01 10.2,21.01 | 10.2,21.01 10.2,20.78 10.79,20.19 v10.79,17.78
TX  (via drill 0.3)
  Top 0.203: v8.38,18.54 8.26,18.41 6.6,18.41 5.97,19.05 3.56,19.05 3.3,19.3 3.3,20.7 3.81,21.21 v3.81,22.23
  Bottom 0.203: v8.38,18.54 8.13,18.29 8.13,17.91 7.11,16.89 5.38,16.89 U3.12 | v3.81,22.23 3.17,22.23 JP1.3
USB_DISC  (via drill 0.3)
  Top 0.203: R7.2 R4.1 4.19,30.86 3.3,29.97 2.67,29.97 2.54,29.84 2.54,23.75 v2.79,23.5
  Bottom 0.203: U3.21 7.23,22.48 5.08,22.48 4.7,22.86 3.3,22.86 2.79,23.37 v2.79,23.5
USBM  (via drill 0.3)
  Top 0.203: 12.95,26.42 R6.1 12.91,26.33 14.35,24.89 14.48,24.89 15.37,24 v15.37,23.37
  Bottom 0.203: v15.37,23.37 14.73,22.73 14.73,21.46 14.35,21.08 14.35,20.91 U3.32
USBP  (via drill 0.3)
  Top 0.203: v15.11,20.95 15.24,21.08 15.24,22.61 14.99,22.86 13.84,22.86 12.91,23.79 R5.1
  Bottom 0.203: U3.33 v15.1,20.95 v15.11,20.95
UVCC  (via drill 0.3)
  Top 0.356: v10.41,30.23 11.3,30.23 11.46,30.07 X1.VBUS
  Bottom 0.203: F1.1 8.91,31.83 7.83,31.83 R1.2
  Bottom 0.356: v10.41,30.23 9.4,30.23 9.27,30.36 F1.1
VDDA  (via drill 0.3)
  Top 0.203: v13.21,18.67 13.59,19.05 16.76,19.05 17.4,19.68 17.4,23.24 v16.89,23.75
  Bottom 0.203: v16.89,23.75 17.27,24.13 JP2.3 | C13.1 5.46,14.85 U3.9 6.87,16.26 6.99,16.26 8.13,17.4 9.14,17.4 10.29,16.26 11.05,16.26 12.95,18.16 12.95,18.41 v13.21,18.67
  Bottom 0.254: C12.A 17.15,31.37 15.75,29.97 15.75,27.22 L2.2 16.76,23.88 v16.89,23.75
WIFI_CS  (via drill 0.3)
  Top 0.203: v12.83,22.99 12.91,22.9 R9.1 12.91,20.16 U2.SPI_CS
  Bottom 0.203: 11.38,22.91 U3.25 11.73,23.24 12.57,23.24 v12.83,22.99
WIFI_EN  (via drill 0.3)
  Top 0.203: 4.33,9.65 U2.VBAT_SW_EN 5.61,9.67 6.22,10.29 8.89,10.29 10.03,11.43 10.03,14.1 v9.65,14.48
  Bottom 0.203: U3.45 12.06,14.11 12.06,14.48 12.19,14.61 12.19,15.11 11.81,15.49 10.67,15.49 v9.65,14.48
WIFI_INT  (via drill 0.3)
  Top 0.203: U2.SPI_IRQ 10.76,19.27 v10.16,18.67
  Bottom 0.203: U3.22 8.64,21.78 8.64,21.49 8.41,21.26 8.41,20.47 9.53,19.36 9.53,18.92 9.78,18.67 v10.16,18.67

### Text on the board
tPlace: VCC | 2 | 1 | PWR | RAW | RST | RST | BTN | GND | VDDA | TX | GND | RX | D7 | A7 | D6 | A6 | D5 | A5 | D4 | A4 | D3 | A3 | D2 | A2 | D1 | A1 | D0 | A0

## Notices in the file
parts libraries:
SparkFun-RF: Licensing: CC v3.0 Share-Alike You are welcome to use this library for commercial purposes.
